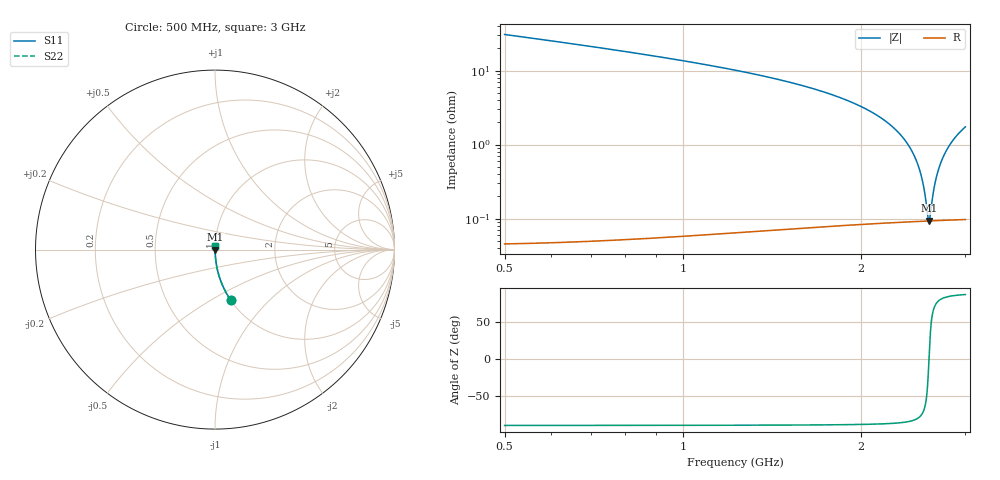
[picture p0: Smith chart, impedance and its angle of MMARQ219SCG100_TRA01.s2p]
! MMARQ219SCG100_TRA01  S-PARAMETER MODEL  ( General Type )
! Model Generated by TAIYO YUDEN Corporation (http://www.ty-top.com)
! Version 1.0
! TAIYO YUDEN Control No. 150609
! Copyright(c) 2015 TAIYO YUDEN CO.,LTD. All Rights Reserved.
! Product Description (link to TY-COMPAS)
! https://ds.yuden.co.jp/TYCOMPAS/or/detail?pn=MMARQ219SCG100JTRA01&u=M
! Products Name : Multilayer Ceramic Capacitors
! Characteristics :
!  Capacitance : 10 pF , Rated Voltage : 250V , TCC : CG / C0G
!  Case Size : 2.0 x 1.25 / 0.079 x 0.049 [mm/inch] , Thickness : 0.85 / 0.033 [mm/inch]
!  (Conditions: Temperature = 25 degC , DC Bias Current/Voltage = 0A / 0V)
! External Node Assignments :
!  1  o---| |---o  2
! GND o---------o GND
! Frequency Range : 500MHz  -  3GHz  [ 401 STEP ]
# MHz S RI R 50
! Freq[MHz].  S11 Real  S11 Imag  S21 Real  S21 Imag  S12 Real  S12 Imag  S22 Real  S22 Imag
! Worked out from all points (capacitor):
!   401 points, 500 MHz to 3 GHz, reference 50 ohm
!   read as one part in series: C = 9.99 pF near 512.5 MHz
!   lowest |Z| = 93.4 mohm at 2.606 GHz (marker M1)
!   series resonance near 2.604 GHz, so ESL is about 370 pH
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500  0.0865 -0.2804  0.9135 0.2804  0.9135 0.2804  0.0865 -0.2804
918.75  0.023 -0.1482  0.977 0.1482  0.977 0.1482  0.023 -0.1482
1337.5  0.00827 -0.0868  0.9917 0.0868  0.9917 0.0868  0.00827 -0.0868
1750  0.00325 -0.0496  0.9968 0.0496  0.9968 0.0496  0.00325 -0.0496
1987.5  0.00194 -0.0333  0.9981 0.0333  0.9981 0.0333  0.00194 -0.0333
2168.75  0.00136 -0.0224  0.9986 0.0224  0.9986 0.0224  0.00136 -0.0224
2337.5  0.00106 -0.0132  0.9989 0.0132  0.9989 0.0132  0.00106 -0.0132
2456.25  0.000958 -0.00712  0.999 0.00712  0.999 0.00712  0.000958 -0.00712
2500  0.000938 -0.00497  0.9991 0.00497  0.9991 0.00497  0.000938 -0.00497
2531.25  0.00093 -0.00345  0.9991 0.00345  0.9991 0.00345  0.00093 -0.00345
2556.25  0.000926 -0.00226  0.9991 0.00226  0.9991 0.00226  0.000926 -0.00226
2587.5  0.000925 -0.000777  0.9991 0.000777  0.9991 0.000777  0.000925 -0.000777
2600  0.000926 -0.00019  0.9991 0.00019  0.9991 0.00019  0.000926 -0.00019
2606.25  0.000927 0.000103  0.9991 -0.000103  0.9991 -0.000103  0.000927 0.000103
2618.75  0.000929 0.000685  0.9991 -0.000685  0.9991 -0.000685  0.000929 0.000685
2643.75  0.000935 0.00184  0.9991 -0.00184  0.9991 -0.00184  0.000935 0.00184
2668.75  0.000944 0.00299  0.9991 -0.00299  0.9991 -0.00299  0.000944 0.00299
2700  0.000958 0.00441  0.999 -0.00441  0.999 -0.00441  0.000958 0.00441
2737.5  0.00098 0.00609  0.999 -0.00609  0.999 -0.00609  0.00098 0.00609
2787.5  0.00102 0.00829  0.999 -0.00829  0.999 -0.00829  0.00102 0.00829
2850  0.00108 0.011  0.9989 -0.011  0.9989 -0.011  0.00108 0.011
3000  0.00127 0.0173  0.9987 -0.0173  0.9987 -0.0173  0.00127 0.0173
